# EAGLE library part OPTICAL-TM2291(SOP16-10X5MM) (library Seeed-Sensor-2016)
314020020
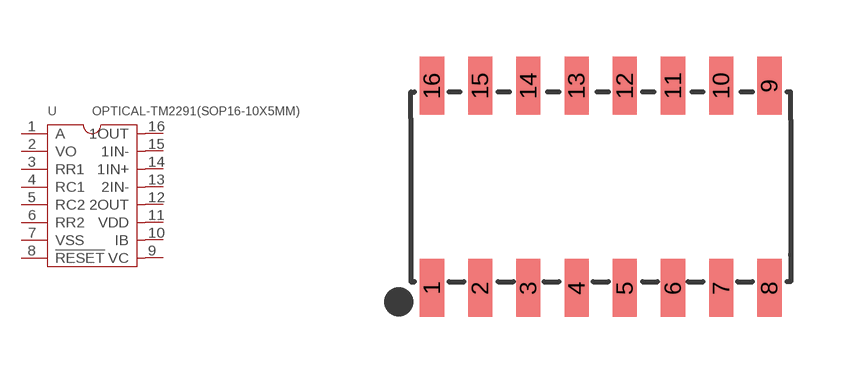
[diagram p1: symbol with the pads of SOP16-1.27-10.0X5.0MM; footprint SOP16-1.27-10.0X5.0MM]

Designator prefix U

## OPTICAL-TM2291(SOP16-10X5MM) (MPN: TM2291; VALUE: TM2291)  [SOP16-1.27-10.0X5.0MM]
1  A
2  VO
3  RR1
4  RC1
5  RC2
6  RR2
7  VSS  sup
8  !RESET  in
9  VC
10  IB
11  VDD  sup
12  2OUT  out
13  2IN-  in
14  1IN+  in
15  1IN-  in
16  1OUT  out

## Footprint SOP16-1.27-10.0X5.0MM (pad centres in mm)
smd 0.635 x 1.524: 1 -4.445,-2.667; 2 -3.175,-2.667; 3 -1.905,-2.667; 4 -0.635,-2.667; 5 0.635,-2.667; 6 1.905,-2.667; 7 3.175,-2.667; 8 4.445,-2.667; 9 4.445,2.667; 10 3.175,2.667; 11 1.905,2.667; 12 0.635,2.667; 13 -0.635,2.667; 14 -1.905,2.667; 15 -3.175,2.667; 16 -4.445,2.667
